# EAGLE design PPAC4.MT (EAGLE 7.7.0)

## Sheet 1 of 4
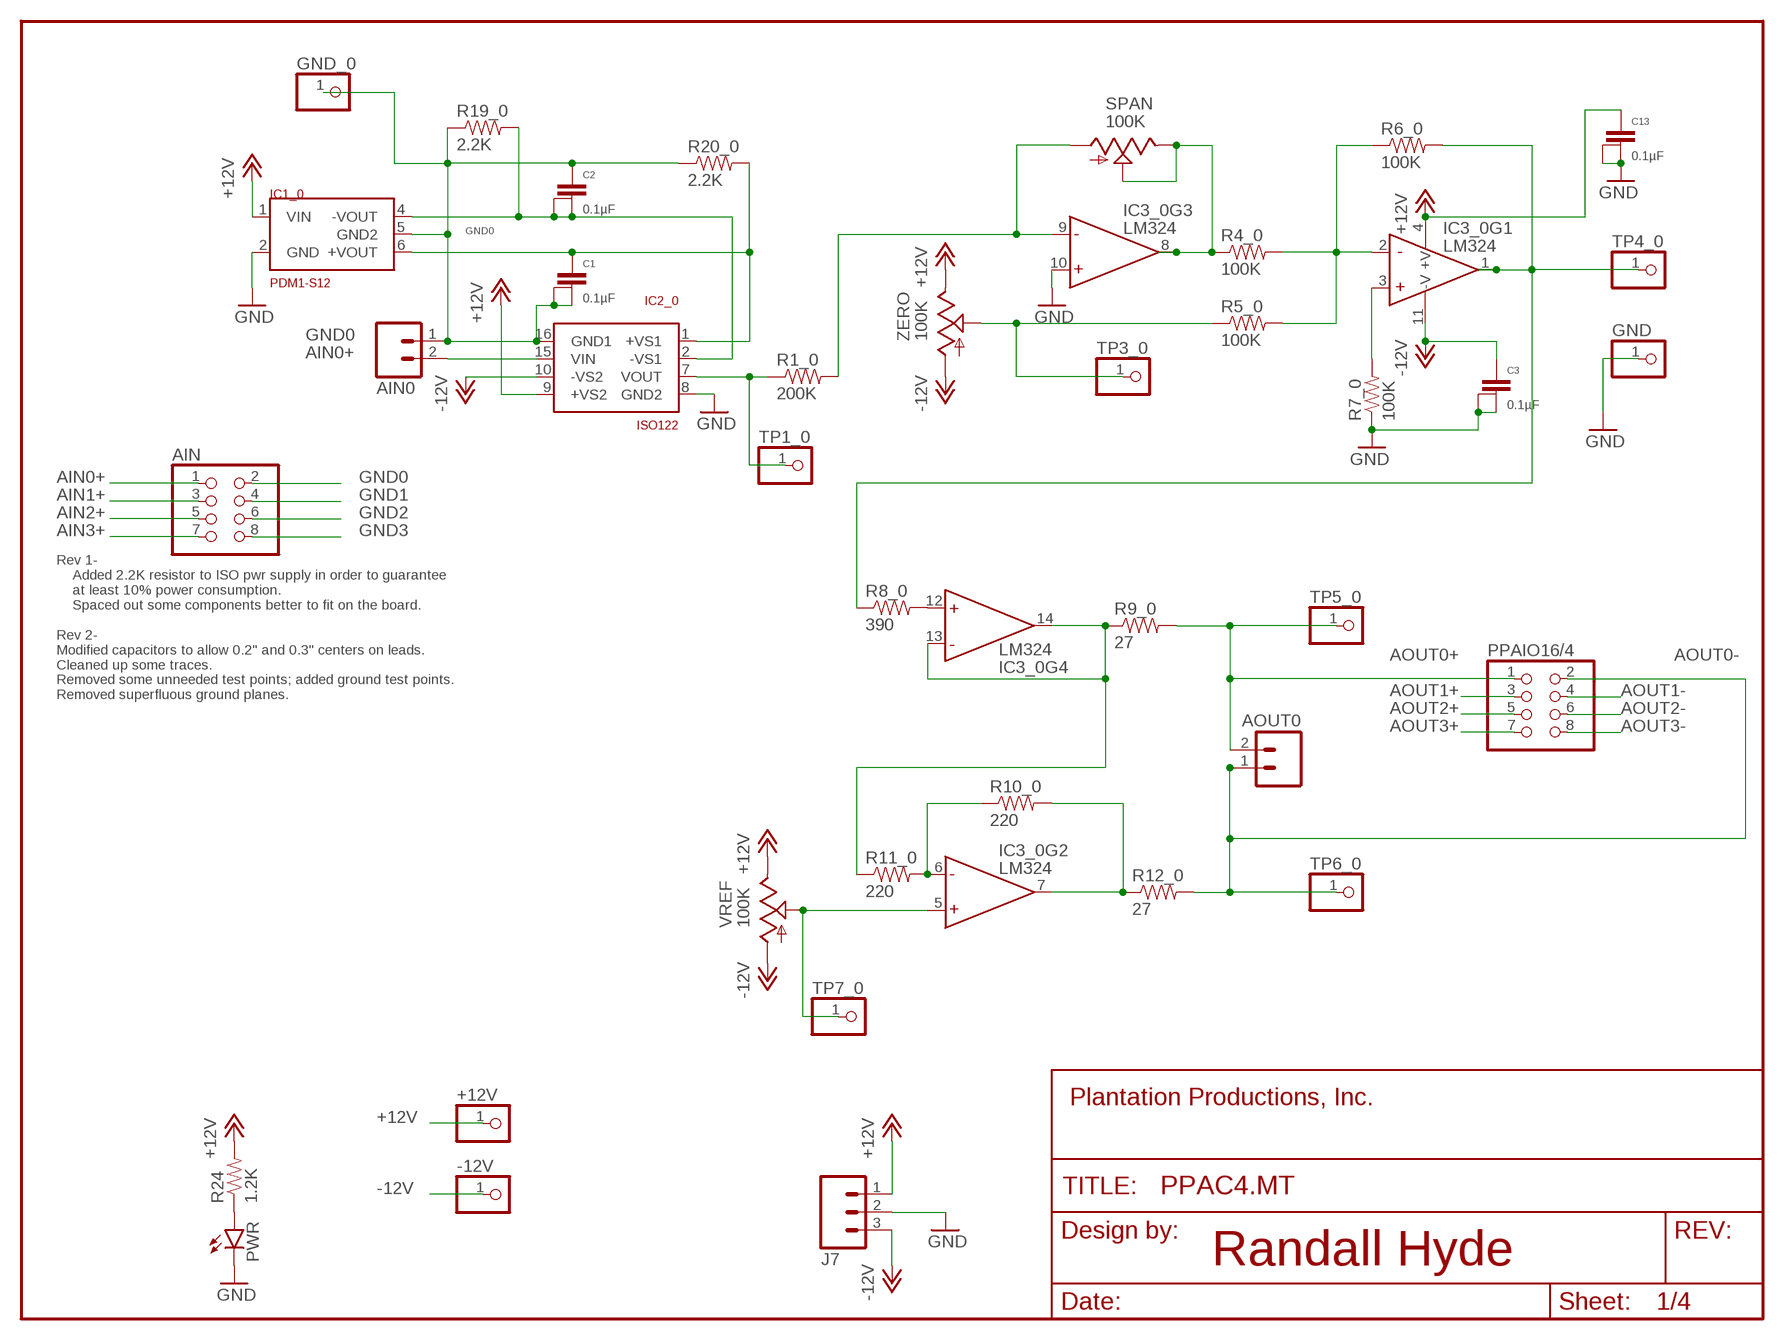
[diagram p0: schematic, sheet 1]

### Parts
+12V  PINHD-1X1  [1X01]
-12V  PINHD-1X1  [1X01]
AIN  PINHD-2X4  [2X04]
AIN0  M025MM  [SCREWTERMINAL-5MM-2]
AOUT0  M025MM  [SCREWTERMINAL-5MM-2]
C1  0.1µF  CAPACITOR  [1+2CAP]
C2  0.1µF  CAPACITOR  [1+2CAP]
C3  0.1µF  CAPACITOR  [1+2CAP]
C13  0.1µF  CAPACITOR  [1+2CAP]
FRAME1  FRAME-LETTERNO_PACKAGE  [DUMMY]
GND  PINHD-1X1  [1X01]
GND_0  PINHD-1X1  [1X01]
IC1_0  PDM1-S12  [SIL6-5]
IC2_0  ISO122  [DIL16-8]
IC3_0  LM324  [DIL14]
J7  M03-SCREW-5MM  [SCREWTERMINAL-5MM-3]
PPAIO16/4  PINHD-2X4  [2X04]
PWR  LED5MM  [LED5MM]
R1_0  200K  10OHM-1/4W-5%(PTH)  [AXIAL-0.3]
R4_0  100K  10OHM-1/4W-5%(PTH)  [AXIAL-0.3]
R5_0  100K  10OHM-1/4W-5%(PTH)  [AXIAL-0.3]
R6_0  100K  10OHM-1/4W-5%(PTH)  [AXIAL-0.3]
R7_0  100K  10OHM-1/4W-5%(PTH)  [AXIAL-0.3]
R8_0  390  10OHM-1/4W-5%(PTH)  [AXIAL-0.3]
R9_0  27  10OHM-1/4W-5%(PTH)  [AXIAL-0.3]
R10_0  220  10OHM-1/4W-5%(PTH)  [AXIAL-0.3]
R11_0  220  10OHM-1/4W-5%(PTH)  [AXIAL-0.3]
R12_0  27  10OHM-1/4W-5%(PTH)  [AXIAL-0.3]
R19_0  2.2K  1KOHM-1/4W-1%(PTH)  [AXIAL-0.3]
R20_0  2.2K  1KOHM-1/4W-1%(PTH)  [AXIAL-0.3]
R24  1.2K  1KOHM-1/4W-1%(PTH)  [AXIAL-0.3]
SPAN  100K  TRIM_US-B64Y  [B64Y]
TP1_0  PINHD-1X1  [1X01]
TP3_0  PINHD-1X1  [1X01]
TP4_0  PINHD-1X1  [1X01]
TP5_0  PINHD-1X1  [1X01]
TP6_0  PINHD-1X1  [1X01]
TP7_0  PINHD-1X1  [1X01]
VREF  100K  TRIM_US-B64Y  [B64Y]
ZERO  100K  TRIM_US-B64Y  [B64Y]

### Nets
+12_0 [RelayConn]: C1.1 IC1_0.6(+VOUT) IC2_0.1(+VS1) R20_0.P$2
+12V: +12V.1 C13.1 IC1_0.1(VIN) IC2_0.9(+VS2) IC3_0.4(+V) J7.1 R24.P$2 VREF.E ZERO.E ; also sheet 2,3,4
-12_0 [RelayConn]: C2.2@1 C2.2@2 IC1_0.4(-VOUT) IC2_0.2(-VS1) R19_0.P$2
-12V [RelayConn]: -12V.1 C3.1 IC2_0.10(-VS2) IC3_0.11(-V) J7.3 VREF.A ZERO.A ; also sheet 2,3,4
AIN0+: AIN0.2 AIN.1 IC2_0.15(VIN)
AIN1+: AIN.3 ; also sheet 2
AIN2+: AIN.5 ; also sheet 3
AIN3+: AIN.7 ; also sheet 4
AOUT0+: AOUT0.2 PPAIO16/4.1 R9_0.P$2 TP5_0.1
AOUT0-: AOUT0.1 PPAIO16/4.2 R12_0.P$2 TP6_0.1
AOUT1+: PPAIO16/4.3 ; also sheet 2
AOUT1-: PPAIO16/4.4 ; also sheet 2
AOUT2+: PPAIO16/4.5 ; also sheet 3
AOUT2-: PPAIO16/4.6 ; also sheet 3
AOUT3+: PPAIO16/4.7 ; also sheet 4
AOUT3-: PPAIO16/4.8 ; also sheet 4
GND [Ground]: C3.2@1 C3.2@2 C13.2@1 C13.2@2 GND.1 IC1_0.2(GND) IC2_0.8(GND2) IC3_0.10(+IN) J7.2 PWR.K(C) R7_0.P$1 ; also sheet 2,3,4
GND0: AIN0.1 AIN.2 C1.2@1 C1.2@2 C2.1 GND_0.1 IC1_0.5(GND2) IC2_0.16(GND1) R19_0.P$1 R20_0.P$1
GND1: AIN.4 ; also sheet 2
GND2: AIN.6 ; also sheet 3
GND3: AIN.8 ; also sheet 4
N$1: IC3_0.9(-IN) R1_0.P$2 SPAN.A
N$2: IC3_0.3(+IN) R7_0.P$2
N$3: IC3_0.8(OUT) R4_0.P$1 SPAN.E SPAN.S
N$4: IC3_0.2(-IN) R4_0.P$2 R5_0.P$2 R6_0.P$1
N$5: IC3_0.1(OUT) R6_0.P$2 R8_0.P$1 TP4_0.1
N$6: R5_0.P$1 TP3_0.1 ZERO.S
N$8: IC2_0.7(VOUT) R1_0.P$1 TP1_0.1
N$9: IC3_0.12(+IN) R8_0.P$2
N$10: IC3_0.7(OUT) R10_0.P$2 R12_0.P$1
N$11: IC3_0.13(-IN) IC3_0.14(OUT) R9_0.P$1 R11_0.P$1
N$12: IC3_0.6(-IN) R10_0.P$1 R11_0.P$2
N$13: IC3_0.5(+IN) TP7_0.1 VREF.S
N$26: PWR.A R24.P$1

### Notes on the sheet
- Rev 1-
      Added 2.2K resistor to ISO pwr supply in order to guarantee
      at least 10% power consumption.
      Spaced out some components better to fit on the board.
  
  Rev 2-
  Modified capacitors to allow 0.2" and 0.3" centers on leads.
  Cleaned up some traces.
  Removed some unneeded test points; added ground test points.
  Removed superfluous ground planes.
- Randall Hyde

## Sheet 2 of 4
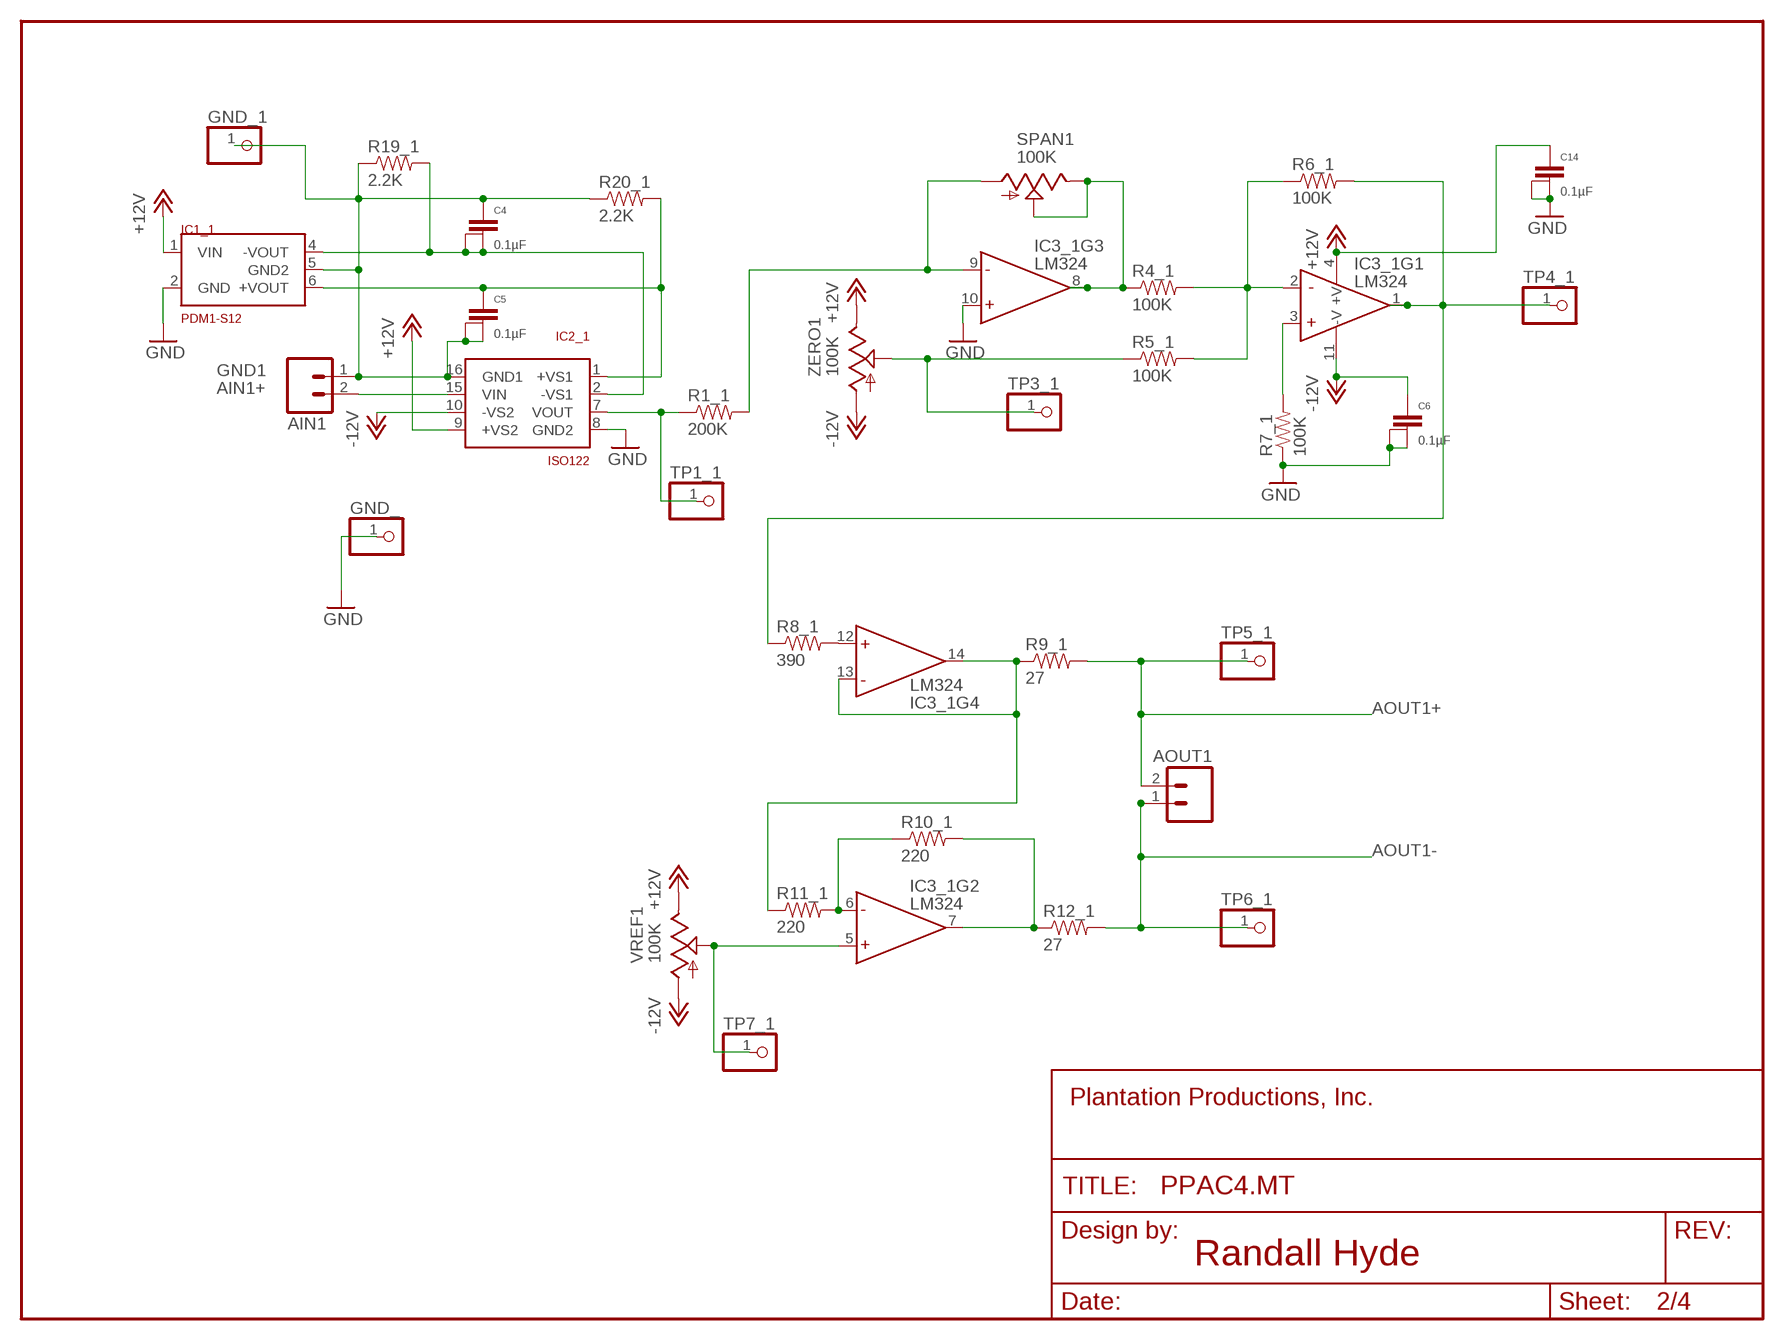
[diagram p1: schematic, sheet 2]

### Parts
AIN1  M025MM  [SCREWTERMINAL-5MM-2]
AOUT1  M025MM  [SCREWTERMINAL-5MM-2]
C4  0.1µF  CAPACITOR  [1+2CAP]
C5  0.1µF  CAPACITOR  [1+2CAP]
C6  0.1µF  CAPACITOR  [1+2CAP]
C14  0.1µF  CAPACITOR  [1+2CAP]
FRAME2  FRAME-LETTERNO_PACKAGE  [DUMMY]
GND_  PINHD-1X1  [1X01]
GND_1  PINHD-1X1  [1X01]
IC1_1  PDM1-S12  [SIL6-5]
IC2_1  ISO122  [DIL16-8]
IC3_1  LM324  [DIL14]
R1_1  200K  10OHM-1/4W-5%(PTH)  [AXIAL-0.3]
R4_1  100K  10OHM-1/4W-5%(PTH)  [AXIAL-0.3]
R5_1  100K  10OHM-1/4W-5%(PTH)  [AXIAL-0.3]
R6_1  100K  10OHM-1/4W-5%(PTH)  [AXIAL-0.3]
R7_1  100K  10OHM-1/4W-5%(PTH)  [AXIAL-0.3]
R8_1  390  10OHM-1/4W-5%(PTH)  [AXIAL-0.3]
R9_1  27  10OHM-1/4W-5%(PTH)  [AXIAL-0.3]
R10_1  220  10OHM-1/4W-5%(PTH)  [AXIAL-0.3]
R11_1  220  10OHM-1/4W-5%(PTH)  [AXIAL-0.3]
R12_1  27  10OHM-1/4W-5%(PTH)  [AXIAL-0.3]
R19_1  2.2K  1KOHM-1/4W-1%(PTH)  [AXIAL-0.3]
R20_1  2.2K  1KOHM-1/4W-1%(PTH)  [AXIAL-0.3]
SPAN1  100K  TRIM_US-B64Y  [B64Y]
TP1_1  PINHD-1X1  [1X01]
TP3_1  PINHD-1X1  [1X01]
TP4_1  PINHD-1X1  [1X01]
TP5_1  PINHD-1X1  [1X01]
TP6_1  PINHD-1X1  [1X01]
TP7_1  PINHD-1X1  [1X01]
VREF1  100K  TRIM_US-B64Y  [B64Y]
ZERO1  100K  TRIM_US-B64Y  [B64Y]

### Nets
+12_1 [RelayConn]: C5.1 IC1_1.6(+VOUT) IC2_1.1(+VS1) R20_1.P$2
+12V: C14.1 IC1_1.1(VIN) IC2_1.9(+VS2) IC3_1.4(+V) VREF1.E ZERO1.E ; also sheet 1,3,4
-12_1 [RelayConn]: C4.2@1 C4.2@2 IC1_1.4(-VOUT) IC2_1.2(-VS1) R19_1.P$2
-12V [RelayConn]: C6.1 IC2_1.10(-VS2) IC3_1.11(-V) VREF1.A ZERO1.A ; also sheet 1,3,4
AIN1+: AIN1.2 IC2_1.15(VIN) ; also sheet 1
AOUT1+: AOUT1.2 R9_1.P$2 TP5_1.1 ; also sheet 1
AOUT1-: AOUT1.1 R12_1.P$2 TP6_1.1 ; also sheet 1
GND [Ground]: C6.2@1 C6.2@2 C14.2@1 C14.2@2 GND_.1 IC1_1.2(GND) IC2_1.8(GND2) IC3_1.10(+IN) R7_1.P$1 ; also sheet 1,3,4
GND1: AIN1.1 C4.1 C5.2@1 C5.2@2 GND_1.1 IC1_1.5(GND2) IC2_1.16(GND1) R19_1.P$1 R20_1.P$1 ; also sheet 1
N$17: IC3_1.9(-IN) R1_1.P$2 SPAN1.A
N$18: IC3_1.8(OUT) R4_1.P$1 SPAN1.E SPAN1.S
N$19: IC3_1.2(-IN) R4_1.P$2 R5_1.P$2 R6_1.P$1
N$20: IC3_1.1(OUT) R6_1.P$2 R8_1.P$1 TP4_1.1
N$22: IC2_1.7(VOUT) R1_1.P$1 TP1_1.1
N$23: R5_1.P$1 TP3_1.1 ZERO1.S
N$24: IC3_1.3(+IN) R7_1.P$2
N$29: IC3_1.7(OUT) R10_1.P$2 R12_1.P$1
N$30: IC3_1.12(+IN) R8_1.P$2
N$31: IC3_1.13(-IN) IC3_1.14(OUT) R9_1.P$1 R11_1.P$1
N$32: IC3_1.6(-IN) R10_1.P$1 R11_1.P$2
N$33: IC3_1.5(+IN) TP7_1.1 VREF1.S

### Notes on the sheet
- Randall Hyde

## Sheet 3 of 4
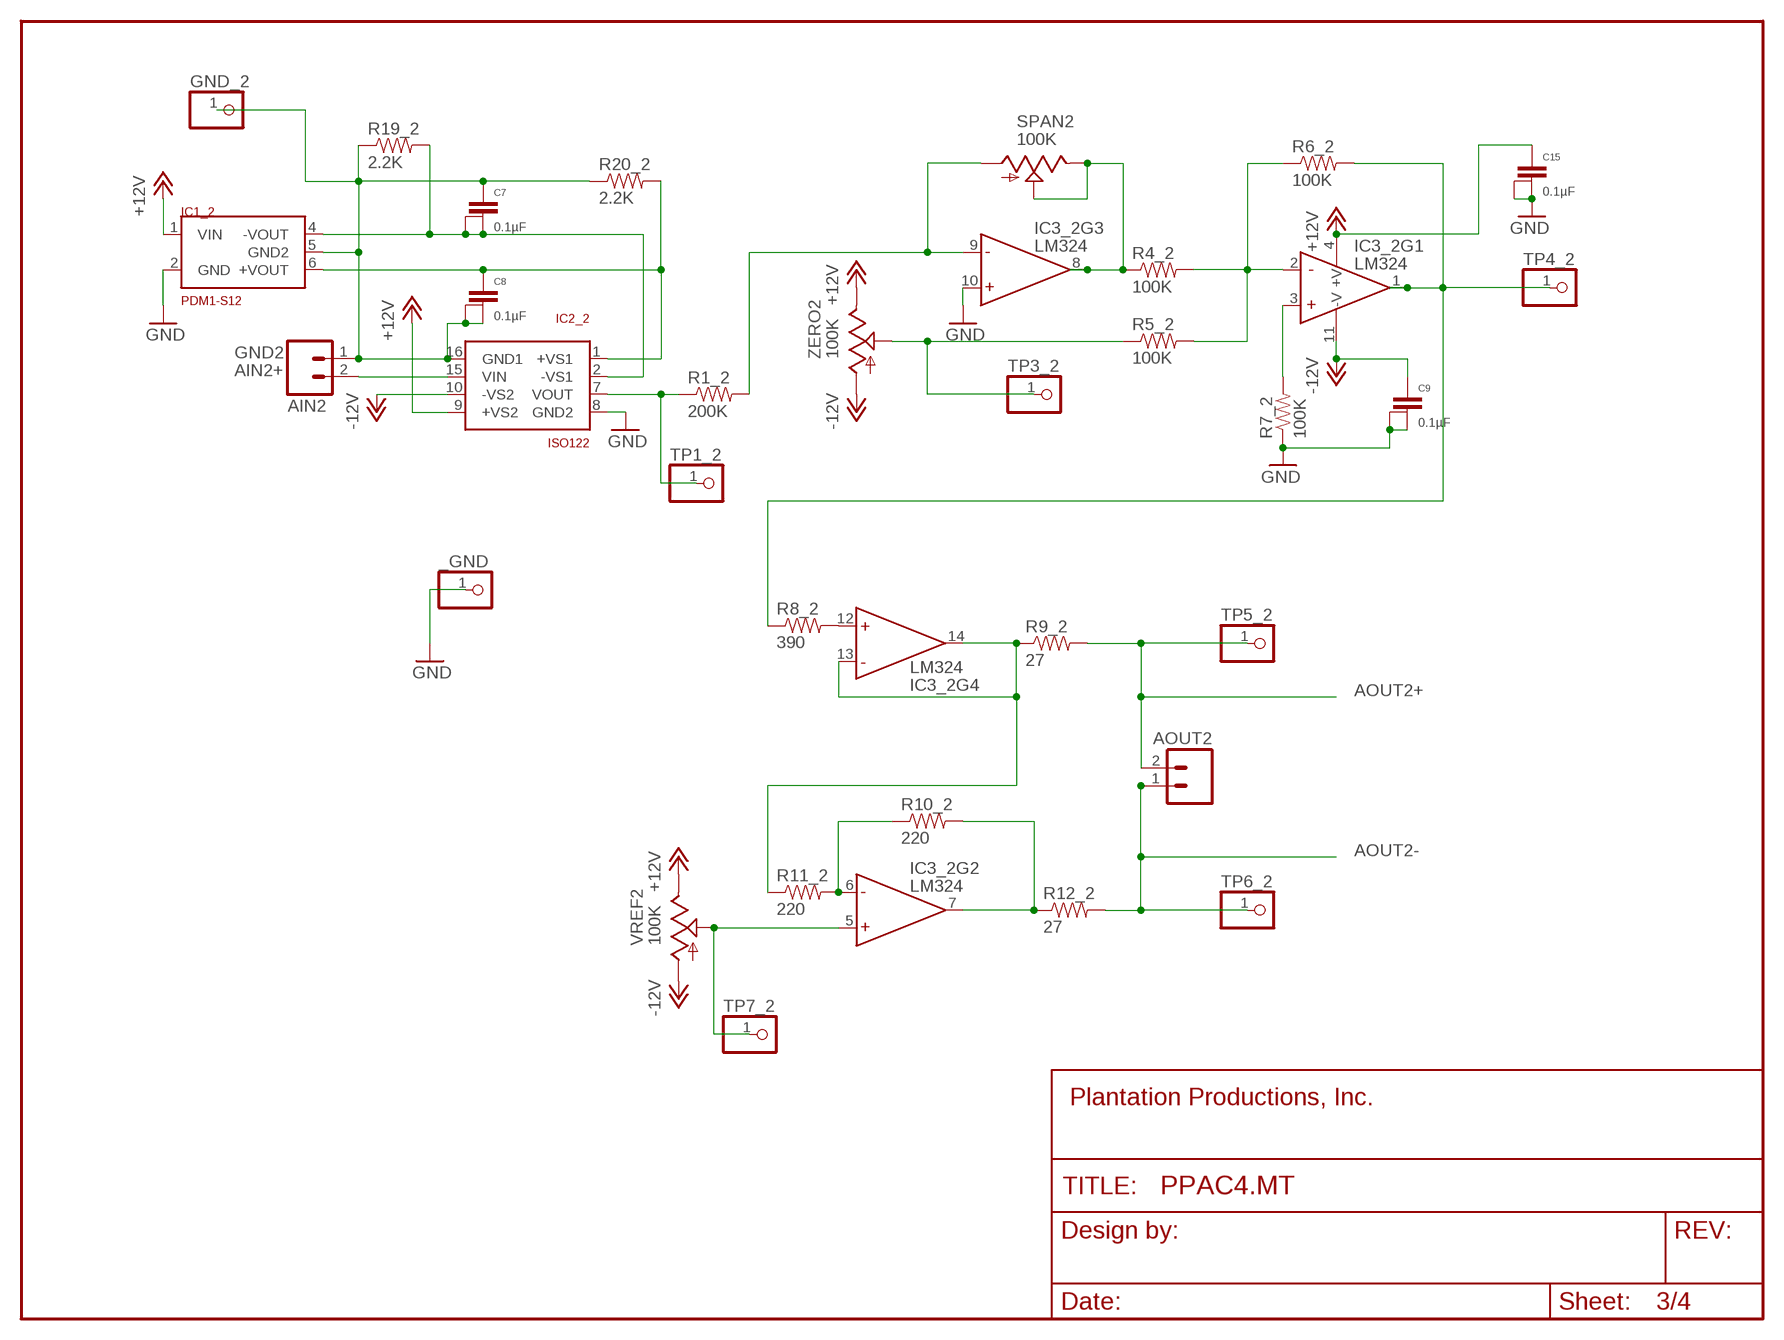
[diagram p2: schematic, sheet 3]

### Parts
_GND  PINHD-1X1  [1X01]
AIN2  M025MM  [SCREWTERMINAL-5MM-2]
AOUT2  M025MM  [SCREWTERMINAL-5MM-2]
C7  0.1µF  CAPACITOR  [1+2CAP]
C8  0.1µF  CAPACITOR  [1+2CAP]
C9  0.1µF  CAPACITOR  [1+2CAP]
C15  0.1µF  CAPACITOR  [1+2CAP]
FRAME3  FRAME-LETTERNO_PACKAGE  [DUMMY]
GND_2  PINHD-1X1  [1X01]
IC1_2  PDM1-S12  [SIL6-5]
IC2_2  ISO122  [DIL16-8]
IC3_2  LM324  [DIL14]
R1_2  200K  10OHM-1/4W-5%(PTH)  [AXIAL-0.3]
R4_2  100K  10OHM-1/4W-5%(PTH)  [AXIAL-0.3]
R5_2  100K  10OHM-1/4W-5%(PTH)  [AXIAL-0.3]
R6_2  100K  10OHM-1/4W-5%(PTH)  [AXIAL-0.3]
R7_2  100K  10OHM-1/4W-5%(PTH)  [AXIAL-0.3]
R8_2  390  10OHM-1/4W-5%(PTH)  [AXIAL-0.3]
R9_2  27  10OHM-1/4W-5%(PTH)  [AXIAL-0.3]
R10_2  220  10OHM-1/4W-5%(PTH)  [AXIAL-0.3]
R11_2  220  10OHM-1/4W-5%(PTH)  [AXIAL-0.3]
R12_2  27  10OHM-1/4W-5%(PTH)  [AXIAL-0.3]
R19_2  2.2K  1KOHM-1/4W-1%(PTH)  [AXIAL-0.3]
R20_2  2.2K  1KOHM-1/4W-1%(PTH)  [AXIAL-0.3]
SPAN2  100K  TRIM_US-B64Y  [B64Y]
TP1_2  PINHD-1X1  [1X01]
TP3_2  PINHD-1X1  [1X01]
TP4_2  PINHD-1X1  [1X01]
TP5_2  PINHD-1X1  [1X01]
TP6_2  PINHD-1X1  [1X01]
TP7_2  PINHD-1X1  [1X01]
VREF2  100K  TRIM_US-B64Y  [B64Y]
ZERO2  100K  TRIM_US-B64Y  [B64Y]

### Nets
+12_2 [RelayConn]: C8.1 IC1_2.6(+VOUT) IC2_2.1(+VS1) R20_2.P$2
+12V: C15.1 IC1_2.1(VIN) IC2_2.9(+VS2) IC3_2.4(+V) VREF2.E ZERO2.E ; also sheet 1,2,4
-12_2 [RelayConn]: C7.2@1 C7.2@2 IC1_2.4(-VOUT) IC2_2.2(-VS1) R19_2.P$2
-12V [RelayConn]: C9.1 IC2_2.10(-VS2) IC3_2.11(-V) VREF2.A ZERO2.A ; also sheet 1,2,4
AIN2+: AIN2.2 IC2_2.15(VIN) ; also sheet 1
AOUT2+: AOUT2.2 R9_2.P$2 TP5_2.1 ; also sheet 1
AOUT2-: AOUT2.1 R12_2.P$2 TP6_2.1 ; also sheet 1
GND [Ground]: _GND.1 C9.2@1 C9.2@2 C15.2@1 C15.2@2 IC1_2.2(GND) IC2_2.8(GND2) IC3_2.10(+IN) R7_2.P$1 ; also sheet 1,2,4
GND2: AIN2.1 C7.1 C8.2@1 C8.2@2 GND_2.1 IC1_2.5(GND2) IC2_2.16(GND1) R19_2.P$1 R20_2.P$1 ; also sheet 1
N$34: IC3_2.9(-IN) R1_2.P$2 SPAN2.A
N$35: IC3_2.8(OUT) R4_2.P$1 SPAN2.E SPAN2.S
N$36: IC3_2.2(-IN) R4_2.P$2 R5_2.P$2 R6_2.P$1
N$37: IC3_2.1(OUT) R6_2.P$2 R8_2.P$1 TP4_2.1
N$39: IC2_2.7(VOUT) R1_2.P$1 TP1_2.1
N$40: R5_2.P$1 TP3_2.1 ZERO2.S
N$41: IC3_2.3(+IN) R7_2.P$2
N$45: IC3_2.7(OUT) R10_2.P$2 R12_2.P$1
N$46: IC3_2.12(+IN) R8_2.P$2
N$47: IC3_2.13(-IN) IC3_2.14(OUT) R9_2.P$1 R11_2.P$1
N$48: IC3_2.6(-IN) R10_2.P$1 R11_2.P$2
N$49: IC3_2.5(+IN) TP7_2.1 VREF2.S

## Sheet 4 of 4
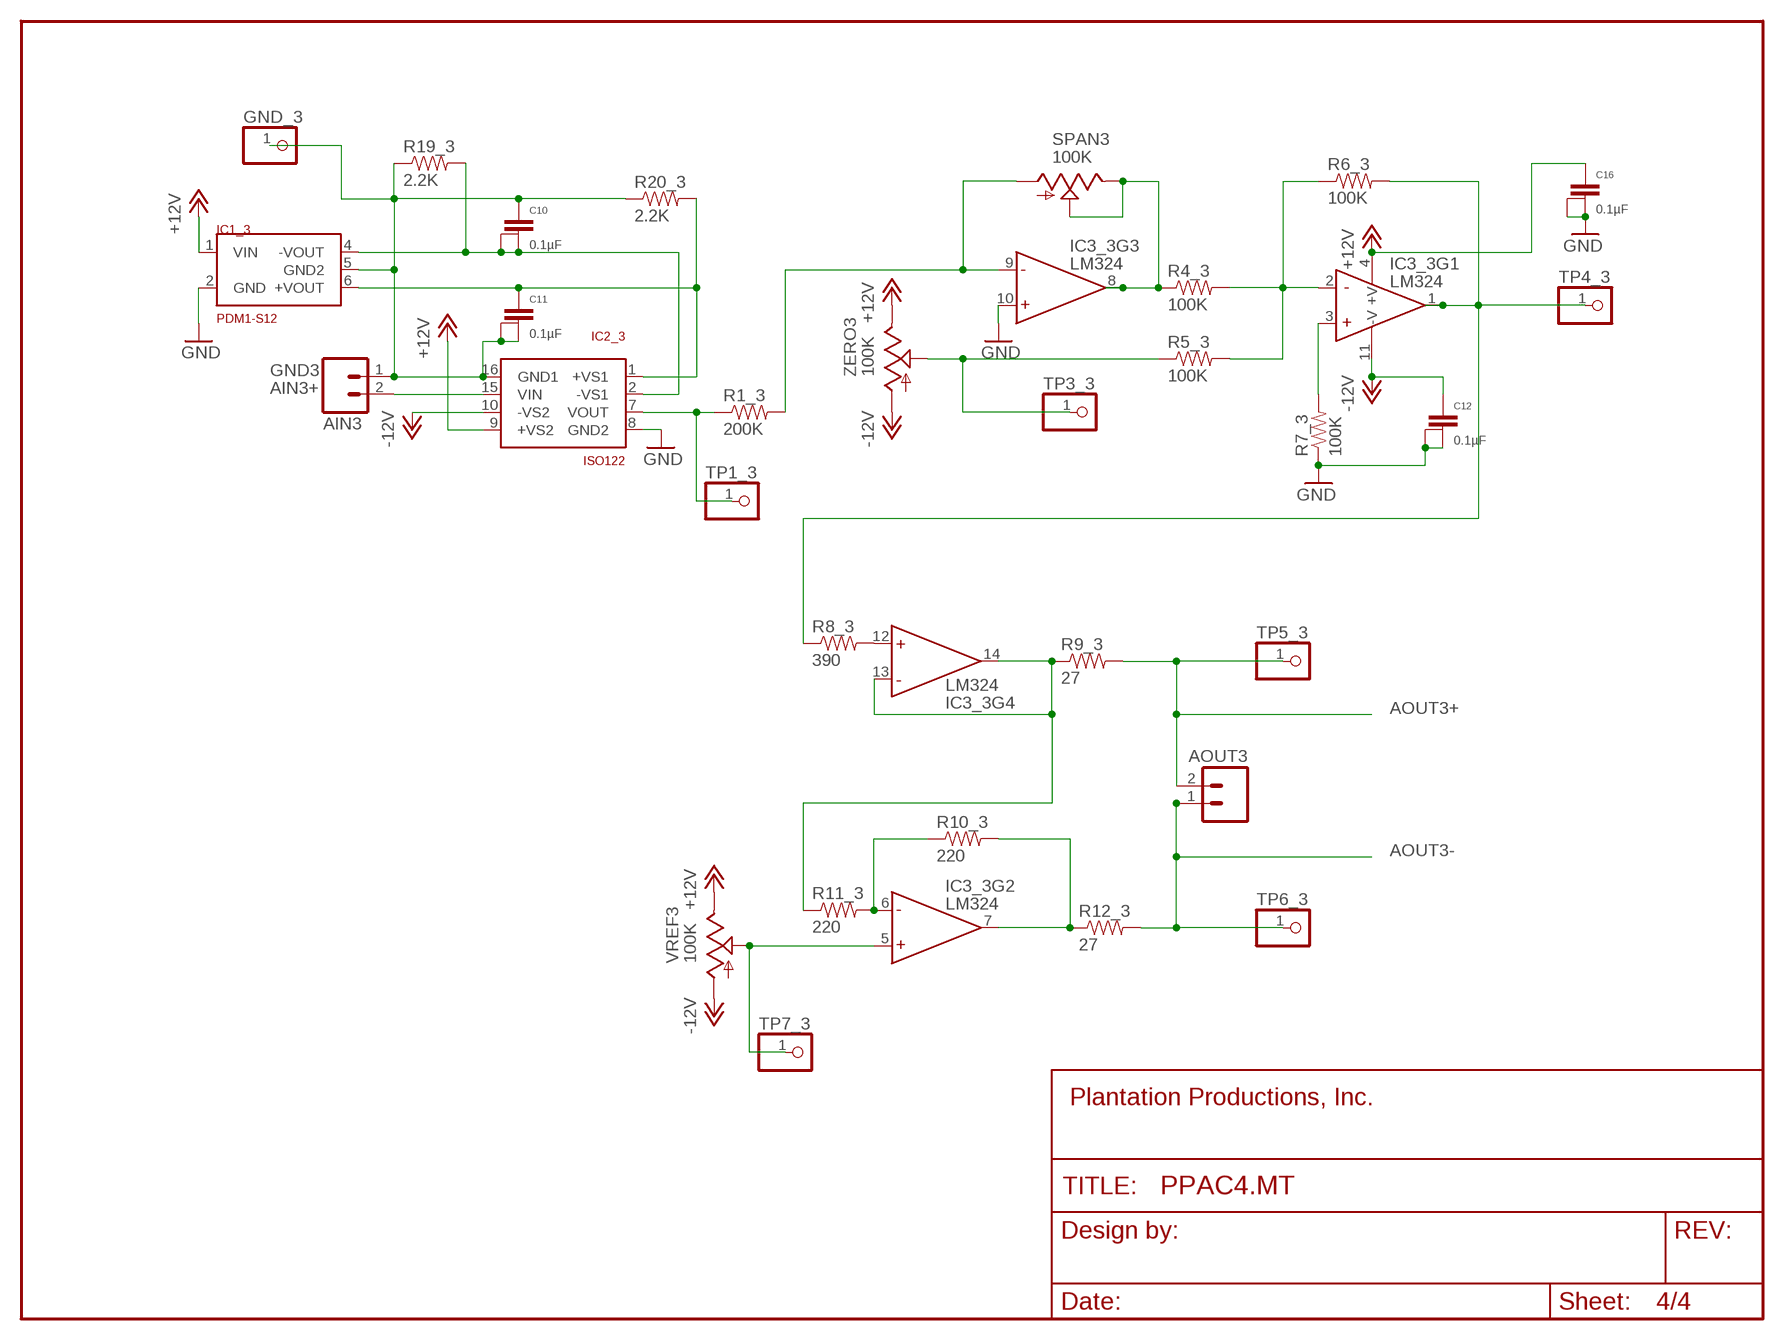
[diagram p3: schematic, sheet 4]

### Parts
AIN3  M025MM  [SCREWTERMINAL-5MM-2]
AOUT3  M025MM  [SCREWTERMINAL-5MM-2]
C10  0.1µF  CAPACITOR  [1+2CAP]
C11  0.1µF  CAPACITOR  [1+2CAP]
C12  0.1µF  CAPACITOR  [1+2CAP]
C16  0.1µF  CAPACITOR  [1+2CAP]
FRAME4  FRAME-LETTERNO_PACKAGE  [DUMMY]
GND_3  PINHD-1X1  [1X01]
IC1_3  PDM1-S12  [SIL6-5]
IC2_3  ISO122  [DIL16-8]
IC3_3  LM324  [DIL14]
R1_3  200K  10OHM-1/4W-5%(PTH)  [AXIAL-0.3]
R4_3  100K  10OHM-1/4W-5%(PTH)  [AXIAL-0.3]
R5_3  100K  10OHM-1/4W-5%(PTH)  [AXIAL-0.3]
R6_3  100K  10OHM-1/4W-5%(PTH)  [AXIAL-0.3]
R7_3  100K  10OHM-1/4W-5%(PTH)  [AXIAL-0.3]
R8_3  390  10OHM-1/4W-5%(PTH)  [AXIAL-0.3]
R9_3  27  10OHM-1/4W-5%(PTH)  [AXIAL-0.3]
R10_3  220  10OHM-1/4W-5%(PTH)  [AXIAL-0.3]
R11_3  220  10OHM-1/4W-5%(PTH)  [AXIAL-0.3]
R12_3  27  10OHM-1/4W-5%(PTH)  [AXIAL-0.3]
R19_3  2.2K  1KOHM-1/4W-1%(PTH)  [AXIAL-0.3]
R20_3  2.2K  1KOHM-1/4W-1%(PTH)  [AXIAL-0.3]
SPAN3  100K  TRIM_US-B64Y  [B64Y]
TP1_3  PINHD-1X1  [1X01]
TP3_3  PINHD-1X1  [1X01]
TP4_3  PINHD-1X1  [1X01]
TP5_3  PINHD-1X1  [1X01]
TP6_3  PINHD-1X1  [1X01]
TP7_3  PINHD-1X1  [1X01]
VREF3  100K  TRIM_US-B64Y  [B64Y]
ZERO3  100K  TRIM_US-B64Y  [B64Y]

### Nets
+12_3 [RelayConn]: C11.1 IC1_3.6(+VOUT) IC2_3.1(+VS1) R20_3.P$2
+12V: C16.1 IC1_3.1(VIN) IC2_3.9(+VS2) IC3_3.4(+V) VREF3.E ZERO3.E ; also sheet 1,2,3
-12_3 [RelayConn]: C10.2@1 C10.2@2 IC1_3.4(-VOUT) IC2_3.2(-VS1) R19_3.P$2
-12V [RelayConn]: C12.1 IC2_3.10(-VS2) IC3_3.11(-V) VREF3.A ZERO3.A ; also sheet 1,2,3
AIN3+: AIN3.2 IC2_3.15(VIN) ; also sheet 1
AOUT3+: AOUT3.2 R9_3.P$2 TP5_3.1 ; also sheet 1
AOUT3-: AOUT3.1 R12_3.P$2 TP6_3.1 ; also sheet 1
GND [Ground]: C12.2@1 C12.2@2 C16.2@1 C16.2@2 IC1_3.2(GND) IC2_3.8(GND2) IC3_3.10(+IN) R7_3.P$1 ; also sheet 1,2,3
GND3: AIN3.1 C10.1 C11.2@1 C11.2@2 GND_3.1 IC1_3.5(GND2) IC2_3.16(GND1) R19_3.P$1 R20_3.P$1 ; also sheet 1
N$50: IC3_3.9(-IN) R1_3.P$2 SPAN3.A
N$51: IC3_3.8(OUT) R4_3.P$1 SPAN3.E SPAN3.S
N$52: IC3_3.2(-IN) R4_3.P$2 R5_3.P$2 R6_3.P$1
N$53: IC3_3.1(OUT) R6_3.P$2 R8_3.P$1 TP4_3.1
N$55: IC2_3.7(VOUT) R1_3.P$1 TP1_3.1
N$56: R5_3.P$1 TP3_3.1 ZERO3.S
N$57: IC3_3.3(+IN) R7_3.P$2
N$61: IC3_3.7(OUT) R10_3.P$2 R12_3.P$1
N$62: IC3_3.12(+IN) R8_3.P$2
N$63: IC3_3.13(-IN) IC3_3.14(OUT) R9_3.P$1 R11_3.P$1
N$64: IC3_3.6(-IN) R10_3.P$1 R11_3.P$2
N$65: IC3_3.5(+IN) TP7_3.1 VREF3.S

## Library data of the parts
+12V -12V _GND GND GND_ GND_0 GND_1-GND_3 TP1_0 TP1_1-TP1_3 TP3_0 TP3_1-TP3_3 TP4_0 TP4_1-TP4_3 TP5_0 TP5_1-TP5_3 TP6_0 TP6_1-TP6_3 TP7_0 TP7_1-TP7_3 = pinhead:PINHD-1X1: PIN HEADER
AIN PPAIO16/4 = pinhead:PINHD-2X4: PIN HEADER
AIN0 AIN1-AIN3 AOUT0 AOUT1-AOUT3 = SparkFun-Connectors:M02: Standard 2-pin 0.1" header. Use with; STOREFRONT_ID: PRT-08432
C1-C16 = PlantProd:CAPACITOR: Capacitor with three terminals to support multiple capacitor sizes.
FRAME1-FRAME4 = SparkFun-Aesthetics:FRAME-LETTER: Schematic Frame; DESIGNER: Nobody; VERSION: v01
IC1_0 IC1_1-IC1_3 = PlantProd:PDM1-S12: PDM1-12S Isolated Power Supply 12V to +/-12V
IC2_0 IC2_1-IC2_3 = PlantProd:ISO122: ISO122 - single channel isolation amplifier
IC3_0 IC3_1-IC3_3 = PlantProd:LM324: LM324 quad op-amp
J7 = SparkFun-Connectors:M03: Header 3 Standard 3-pin 0.1" header. Use with straight break away headers (SKU : PRT-00116), right angle break away headers (PRT-00553), swiss pins (PRT-00743), machine pins (PRT-00117), and female headers (PRT-00115). Molex polarized connector foot print use with SKU : PRT-08232 with associated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; STOREFRONT_ID: PRT-08433
PWR = SparkFun-LED:LED: LEDs
R1_0 R1_1-R1_3 R4_0 R4_1-R4_3 R5_0 R5_1-R5_3 R6_0 R6_1-R6_3 R7_0 R7_1-R7_3 R8_0 R8_1-R8_3 R9_0 R9_1-R9_3 R10_0 R10_1-R10_3 R11_0 R11_1-R11_3 R12_0 R12_1-R12_3 = SparkFun-Resistors:10OHM-1/4W-5%(PTH): RES-10698; PROD_ID: RES-10698; VALUE: 10
R19_0 R19_1-R19_3 R20_0 R20_1-R20_3 R24 = SparkFun-Resistors:1KOHM-1/4W-1%(PTH): RES-12182; PROD_ID: RES-12182; VALUE: 1K
SPAN SPAN1-SPAN3 VREF VREF1-VREF3 ZERO ZERO1-ZERO3 = pot:TRIM_US-: POTENTIOMETER

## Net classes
1 Ground: width 0.762 mm, drill 1 mm, clearance 0.102 mm
2 RelayConn: width 1.016 mm, drill 0.025 mm, clearance 0.508 mm
3 HiCurSignal: width 1.016 mm, drill 0.025 mm, clearance 1.016 mm

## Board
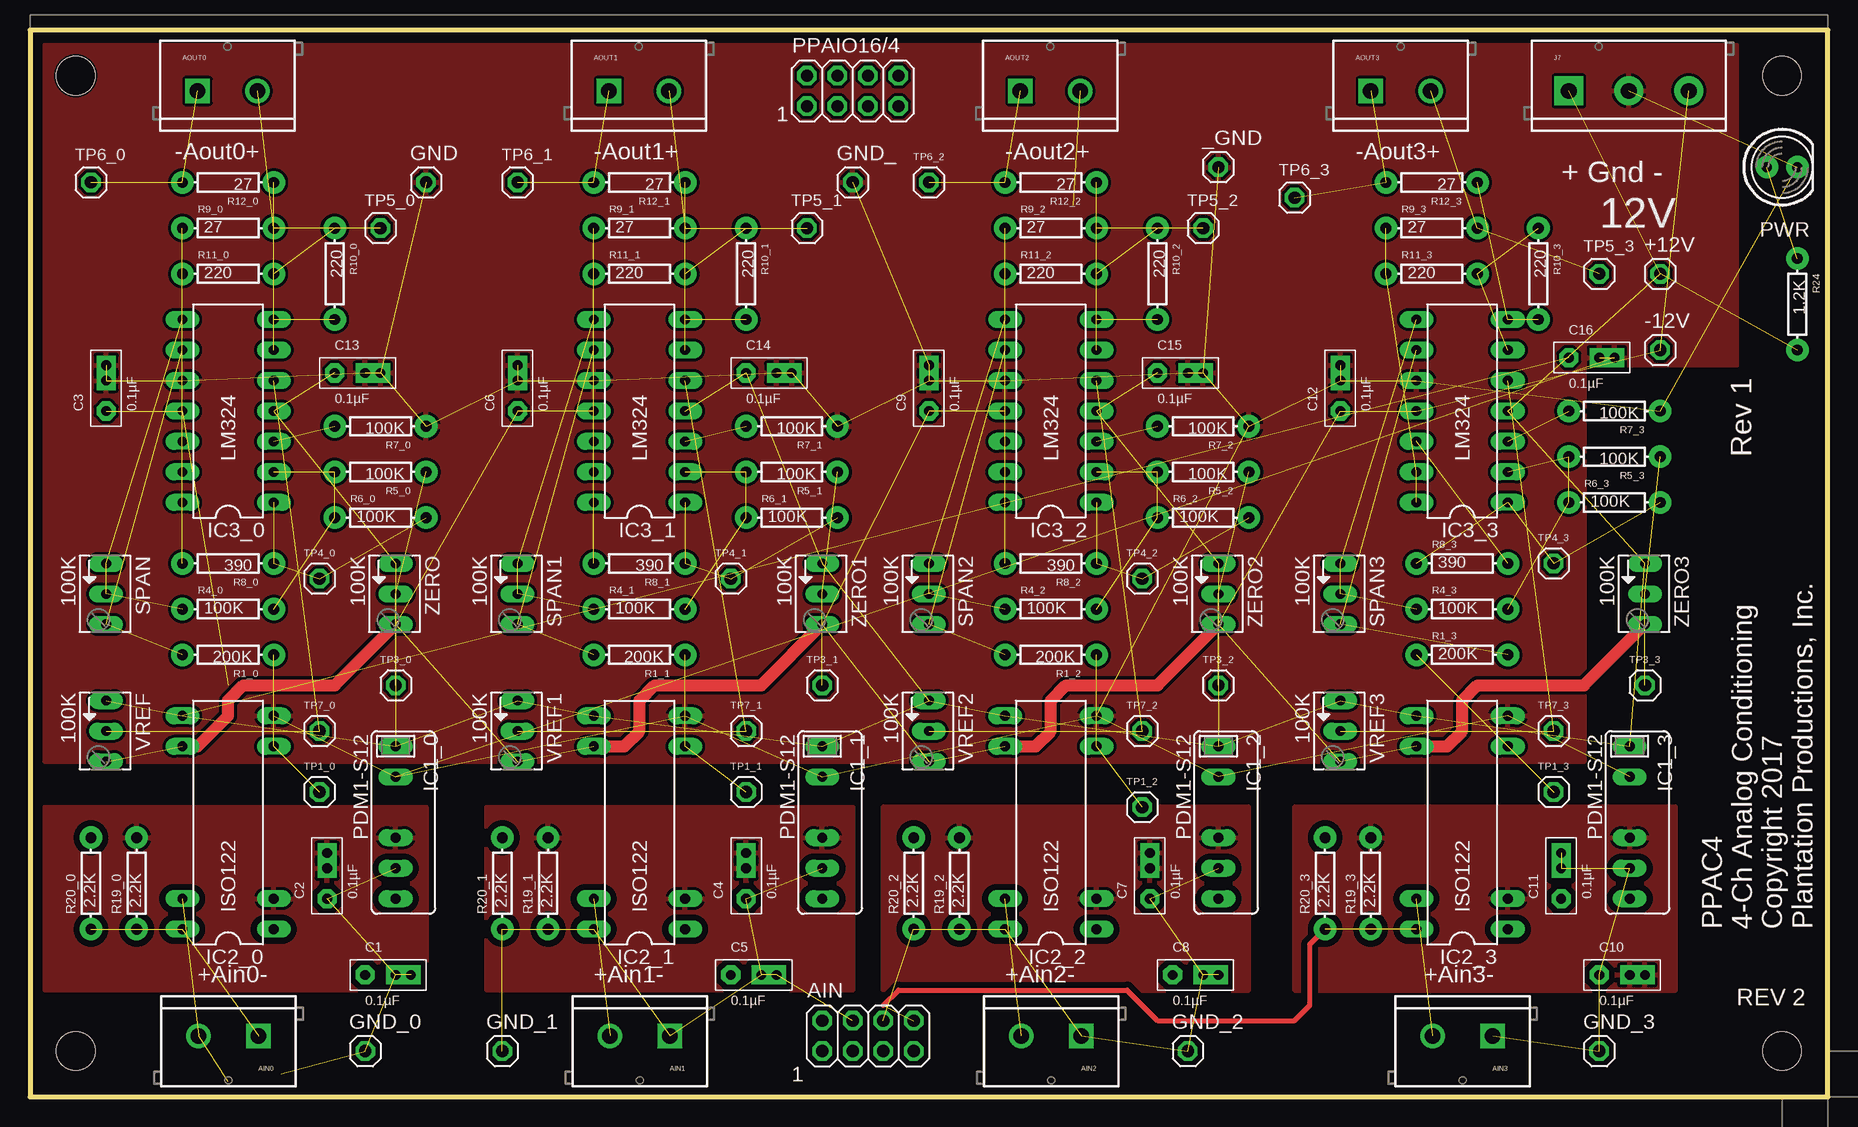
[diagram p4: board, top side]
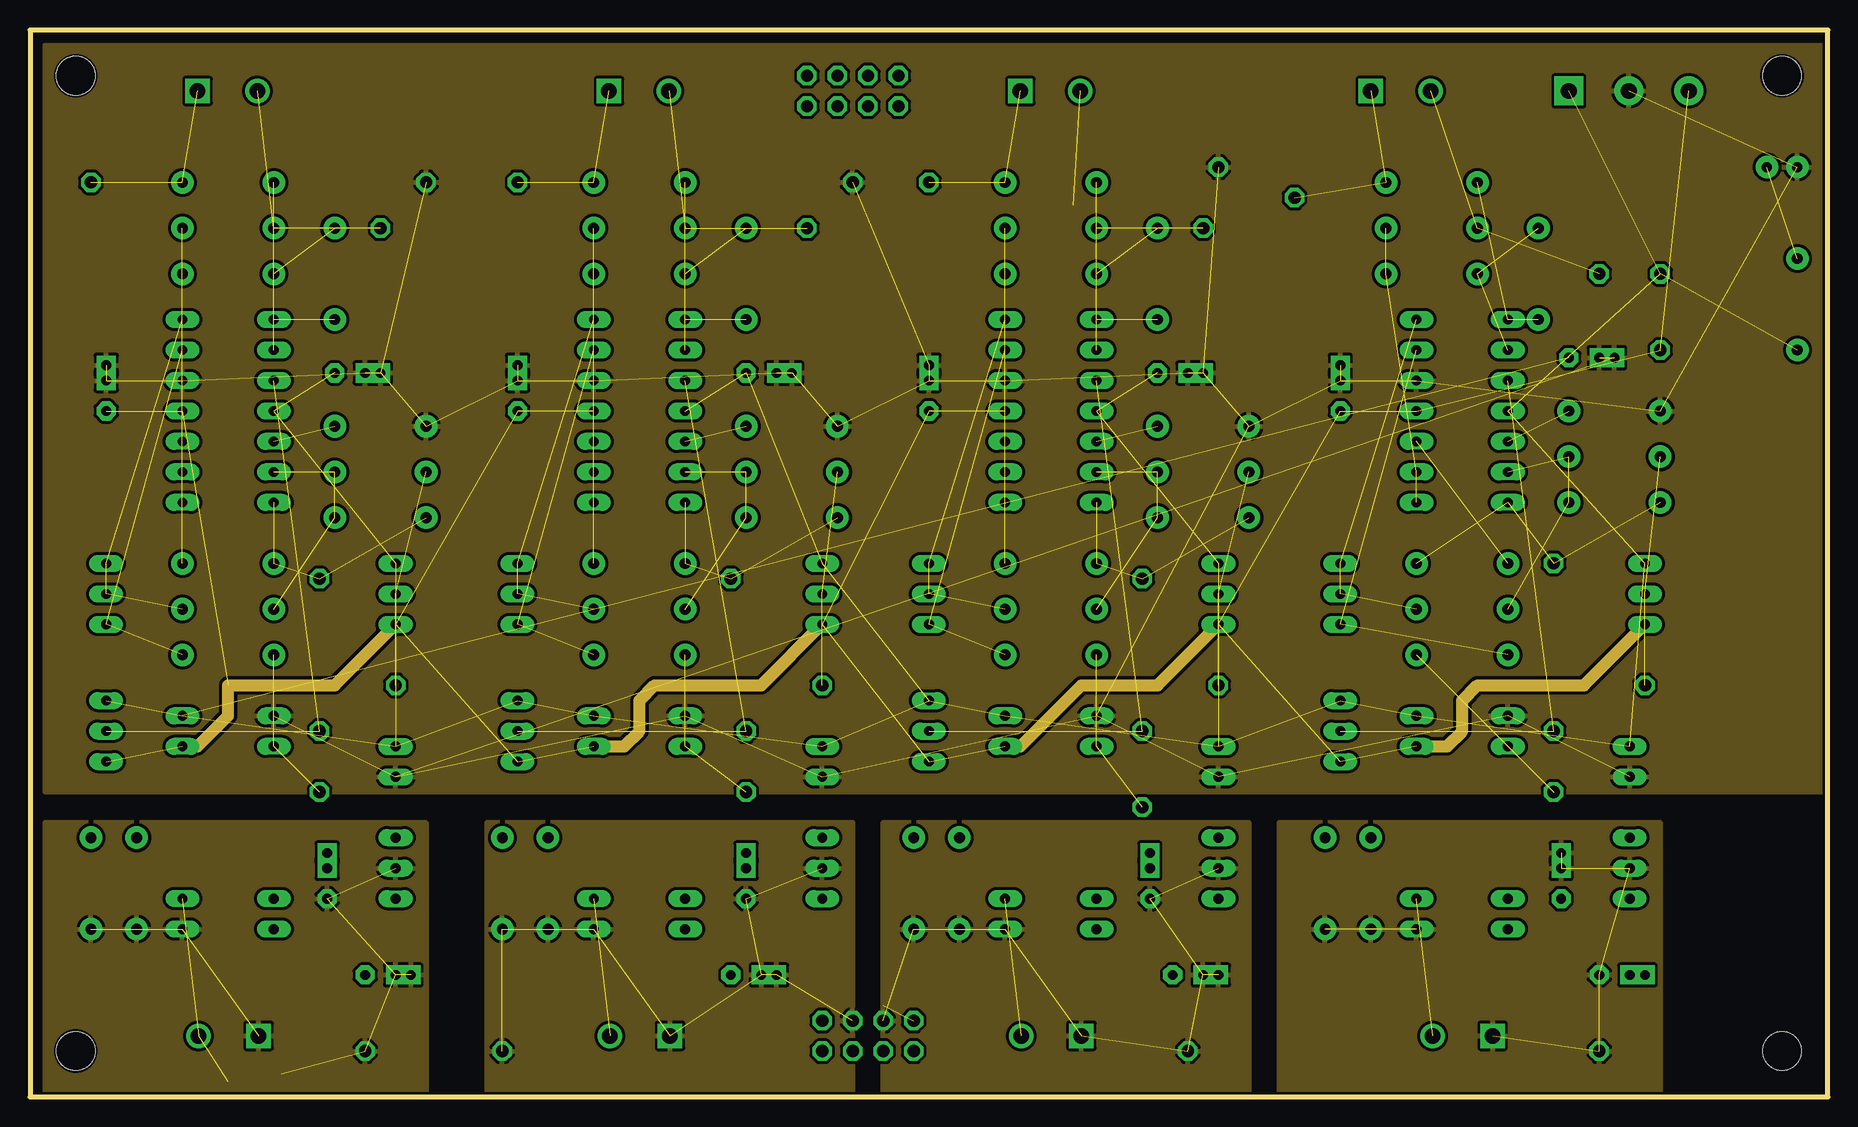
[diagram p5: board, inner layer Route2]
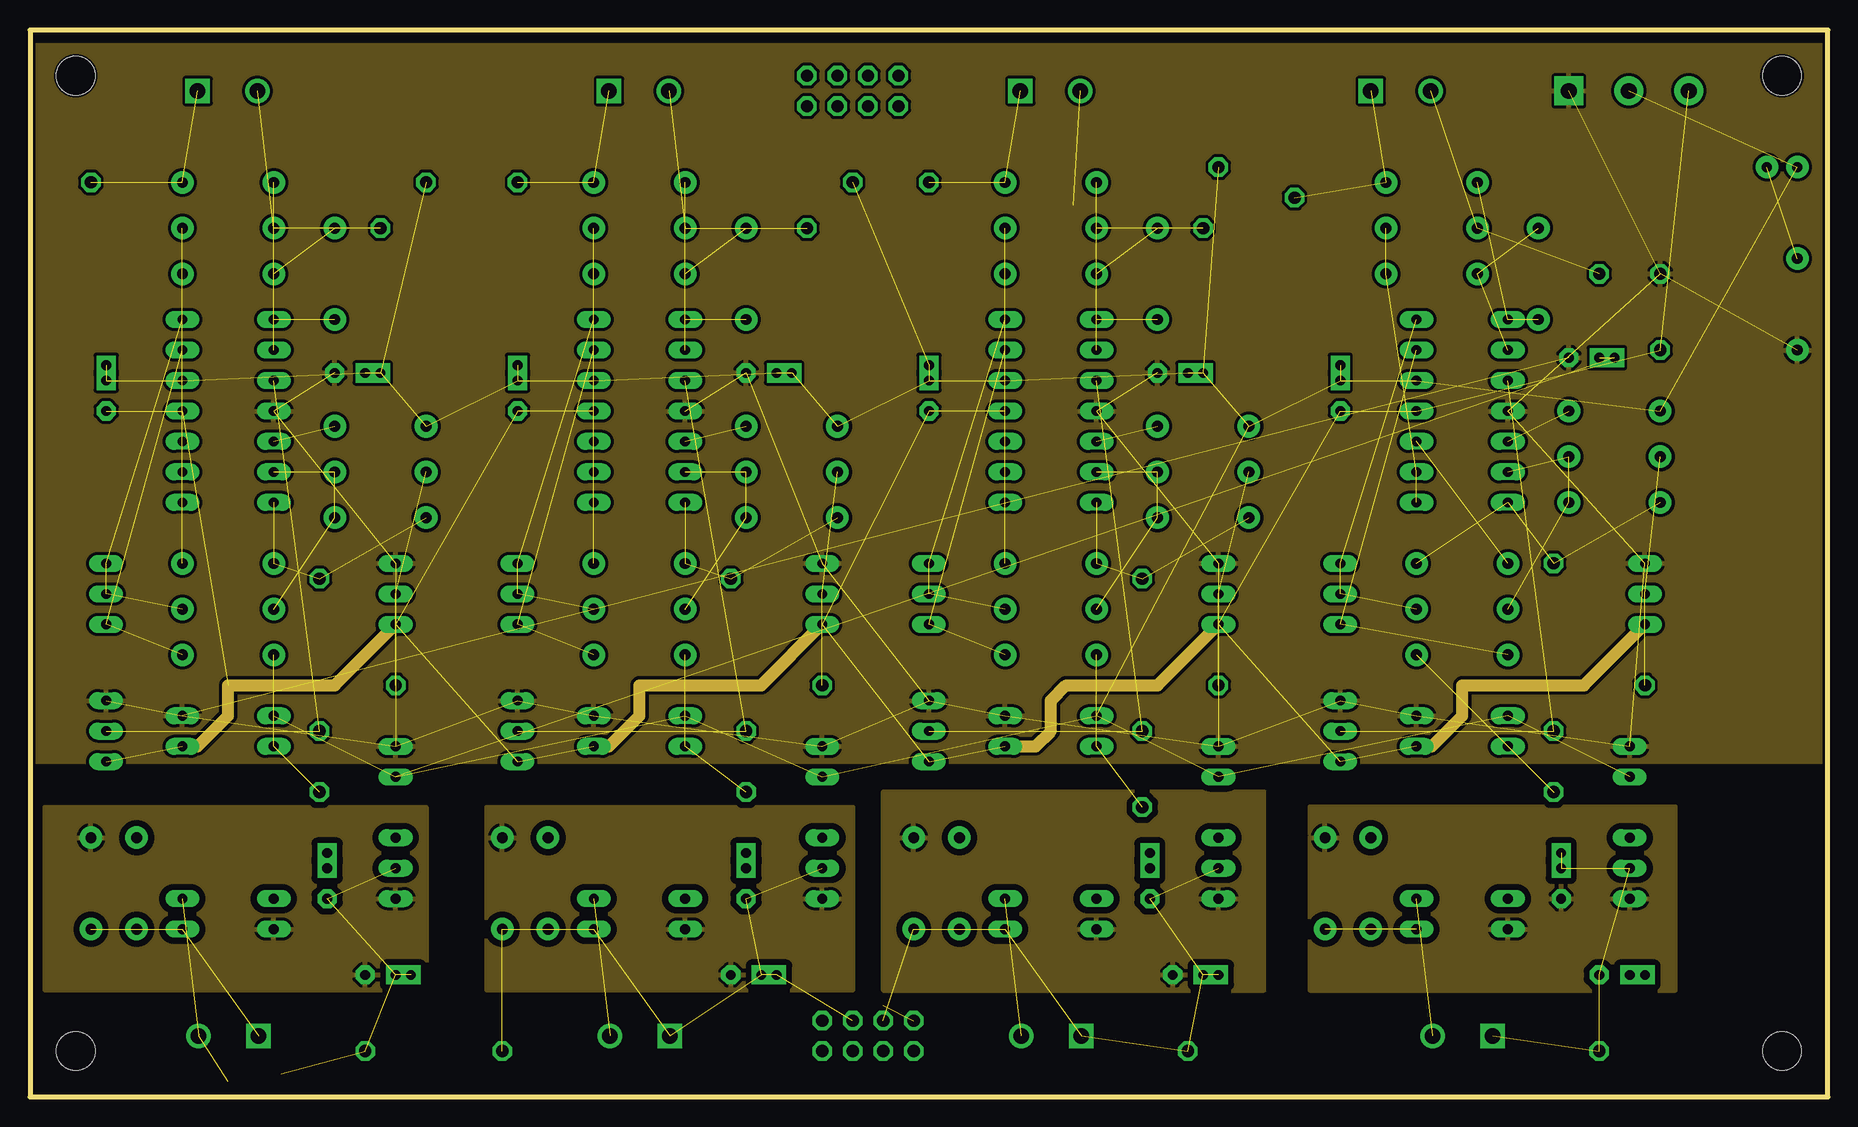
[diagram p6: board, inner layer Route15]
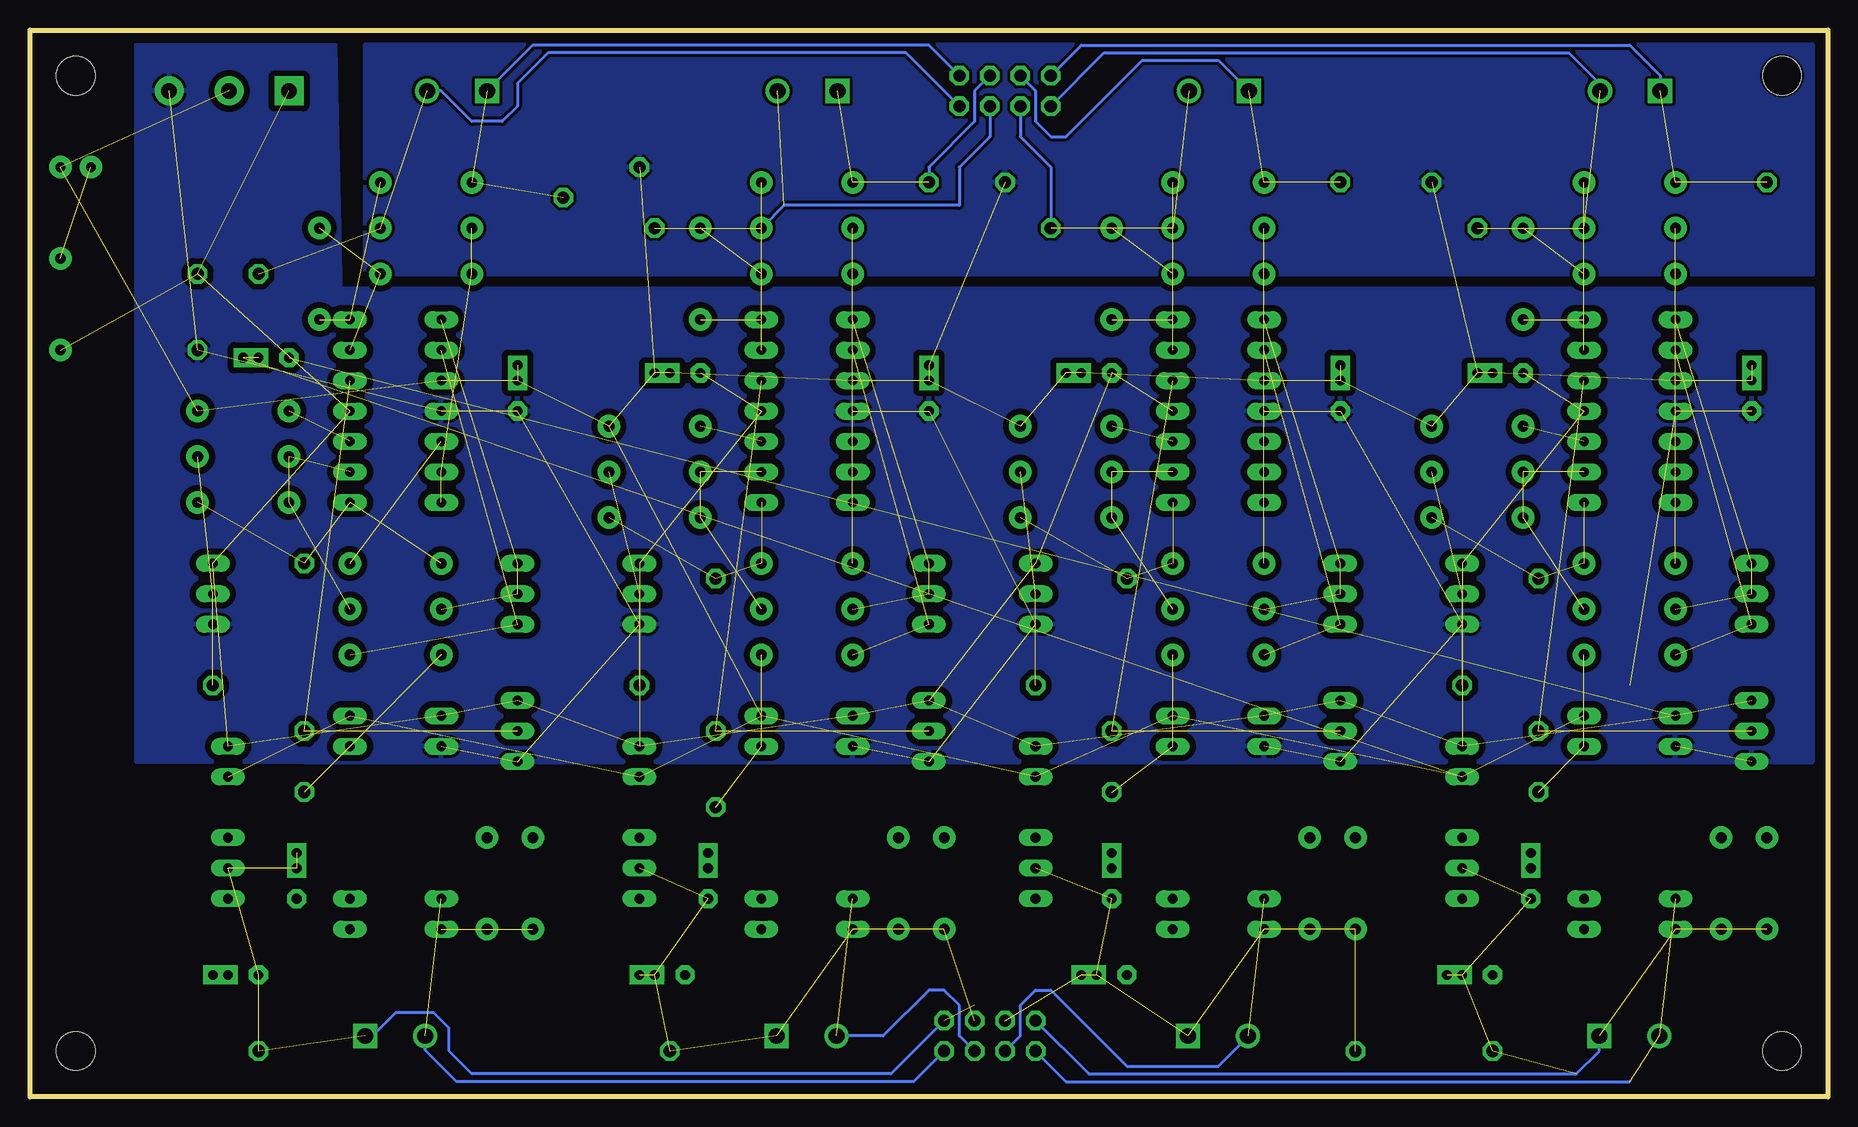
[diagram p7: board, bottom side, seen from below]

Size 149.86 x 88.9 mm. Coordinates in mm from the lower left corner, seen from the top.
Outline: 0,0 149.86,0 149.86,88.9 0,88.9 0,0
Copper layers (1*2*15*16): Top 0.035mm / dielectric 1.5mm / Route2 0.035mm / dielectric 0.15mm / Route15 0.035mm / dielectric 0.2mm / Bottom 0.035mm
Design rules "SeeedStudio_2layer_DRU_no_angle_20140221 *": minimum track width 10mil, minimum drill 20mil, track to track 10mil, track to pad 10mil, pad to pad 10mil, via to via 10mil, smd to smd 8mil, copper to edge 8mil, drill to drill 8mil, minimum pad ring 12mil, minimum via ring 10mil, stop-mask expansion 4mil, vias tented up to drill 25mil, thermal gap 10mil
Holes 3.2 mm at 3.81,85.09 3.81,3.81 146.05,85.09 146.05,3.81

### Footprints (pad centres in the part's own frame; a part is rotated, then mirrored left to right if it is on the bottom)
1X01 = drill 1.016 octagon: 1 0,0
2X04 = drill 1.016 octagon: 1 -3.81,-1.27; 2 -3.81,1.27; 3 -1.27,-1.27; 4 -1.27,1.27; 5 1.27,-1.27; 6 1.27,1.27; 7 3.81,-1.27; 8 3.81,1.27
SCREWTERMINAL-5MM-2 = drill 1.3 pad 2.032 square: 1 0,0 | drill 1.3 pad 2.032: 2 5,0
1+2CAP = drill 0.813 pad 1.6 octagon: 1 -2.54,0 | drill 0.813 pad 1.6 square: 2@1 0,0; 2@2 1.27,0
SIL6-5 = drill 0.813 long: 1 -10.16,0; 2 -7.62,0; 4 -2.54,0; 5 0,0; 6 2.54,0
DIL16-8 = drill 0.813 long: 1 -8.89,-3.81; 2 -6.35,-3.81; 7 6.35,-3.81; 8 8.89,-3.81; 9 8.89,3.81; 10 6.35,3.81; 15 -6.35,3.81; 16 -8.89,3.81
DIL14 = drill 0.813 long: 1 -7.62,-3.81; 2 -5.08,-3.81; 3 -2.54,-3.81; 4 0,-3.81; 5 2.54,-3.81; 6 5.08,-3.81; 7 7.62,-3.81; 8 7.62,3.81; 9 5.08,3.81; 10 2.54,3.81; 11 0,3.81; 12 -2.54,3.81; 13 -5.08,3.81; 14 -7.62,3.81
SCREWTERMINAL-5MM-3 = drill 1.3 pad 2.413 square: 1 0,0 | drill 1.3 pad 2.413: 2 5,0; 3 10,0
LED5MM = drill 0.813 pad 1.88: A -1.27,0; K 1.27,0
AXIAL-0.3 = drill 0.9 pad 1.88: P$1 -3.81,0; P$2 3.81,0
B64Y = drill 0.813 long: A 2.54,0; E -2.54,0; S 0,0

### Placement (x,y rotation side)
+12V  135.89,68.58 0 top
-12V  135.89,62.23 0 top
_GND  99.06,77.47 0 top
AIN  69.85,5.08 0 top
AIN0  19.05,5.08 180 top
AIN1  53.34,5.08 180 top
AIN2  87.63,5.08 180 top
AIN3  121.92,5.08 180 top
AOUT0  13.97,83.82 0 top
AOUT1  48.26,83.82 0 top
AOUT2  82.55,83.82 0 top
AOUT3  111.76,83.82 0 top
C1  30.48,10.16 0 top
C2  24.77,19.05 90 top
C3  6.35,59.69 90 top
C4  59.69,19.05 90 top
C5  60.96,10.16 0 top
C6  40.64,59.69 90 top
C7  93.34,19.05 90 top
C8  97.79,10.16 0 top
C9  74.93,59.69 90 top
C10  133.35,10.16 0 top
C11  127.64,19.05 90 top
C12  109.22,59.69 90 top
C13  27.94,60.33 0 top
C14  62.23,60.33 0 top
C15  96.52,60.33 0 top
C16  130.81,61.59 0 top
FRAME1  114.3,1.27 0 top
FRAME2  114.3,2.54 90 top
FRAME3  not placed on the board
FRAME4  not placed on the board
GND  33.02,76.2 0 top
GND_  68.58,76.2 0 top
GND_0  27.94,3.81 0 top
GND_1  39.37,3.81 0 top
GND_2  96.52,3.81 0 top
GND_3  130.81,3.81 0 top
IC1_0  30.48,19.05 270 top
IC1_1  66.04,19.05 270 top
IC1_2  99.06,19.05 270 top
IC1_3  133.35,19.05 270 top
IC2_0  16.51,22.86 90 top
IC2_1  50.8,22.86 90 top
IC2_2  85.09,22.86 90 top
IC2_3  119.38,22.86 90 top
IC3_0  16.51,57.15 90 top
IC3_1  50.8,57.15 90 top
IC3_2  85.09,57.15 90 top
IC3_3  119.38,57.15 90 top
J7  128.27,83.82 0 top
PPAIO16/4  68.58,83.82 0 top
PWR  146.05,77.47 0 top
R1_0  16.51,36.83 180 top
R1_1  50.8,36.83 180 top
R1_2  85.09,36.83 180 top
R1_3  119.38,36.83 0 top
R4_0  16.51,40.64 0 top
R4_1  50.8,40.64 0 top
R4_2  85.09,40.64 0 top
R4_3  119.38,40.64 0 top
R5_0  29.21,52.07 180 top
R5_1  63.5,52.07 180 top
R5_2  97.79,52.07 180 top
R5_3  132.08,53.34 180 top
R6_0  29.21,48.26 0 top
R6_1  63.5,48.26 0 top
R6_2  97.79,48.26 0 top
R6_3  132.08,49.53 0 top
R7_0  29.21,55.88 180 top
R7_1  63.5,55.88 180 top
R7_2  97.79,55.88 180 top
R7_3  132.08,57.15 180 top
R8_0  16.51,44.45 180 top
R8_1  50.8,44.45 180 top
R8_2  85.09,44.45 180 top
R8_3  119.38,44.45 0 top
R9_0  16.51,72.39 0 top
R9_1  50.8,72.39 0 top
R9_2  85.09,72.39 0 top
R9_3  116.84,72.39 0 top
R10_0  25.4,68.58 270 top
R10_1  59.69,68.58 270 top
R10_2  93.98,68.58 270 top
R10_3  125.73,68.58 270 top
R11_0  16.51,68.58 0 top
R11_1  50.8,68.58 0 top
R11_2  85.09,68.58 0 top
R11_3  116.84,68.58 0 top
R12_0  16.51,76.2 180 top
R12_1  50.8,76.2 180 top
R12_2  85.09,76.2 180 top
R12_3  116.84,76.2 180 top
R19_0  8.89,17.78 90 top
R19_1  43.18,17.78 90 top
R19_2  77.47,17.78 90 top
R19_3  111.76,17.78 90 top
R20_0  5.08,17.78 90 top
R20_1  39.37,17.78 90 top
R20_2  73.66,17.78 90 top
R20_3  107.95,17.78 90 top
R24  147.32,66.04 270 top
SPAN  6.35,41.91 270 top
SPAN1  40.64,41.91 270 top
SPAN2  74.93,41.91 270 top
SPAN3  109.22,41.91 270 top
TP1_0  24.13,25.4 0 top
TP1_1  59.69,25.4 0 top
TP1_2  92.71,24.13 0 top
TP1_3  127,25.4 0 top
TP3_0  30.48,34.29 0 top
TP3_1  66.04,34.29 0 top
TP3_2  99.06,34.29 0 top
TP3_3  134.62,34.29 0 top
TP4_0  24.13,43.18 0 top
TP4_1  58.42,43.18 0 top
TP4_2  92.71,43.18 0 top
TP4_3  127,44.45 0 top
TP5_0  29.21,72.39 0 top
TP5_1  64.77,72.39 0 top
TP5_2  97.79,72.39 0 top
TP5_3  130.81,68.58 0 top
TP6_0  5.08,76.2 0 top
TP6_1  40.64,76.2 0 top
TP6_2  74.93,76.2 0 top
TP6_3  105.41,74.93 0 top
TP7_0  24.13,30.48 0 top
TP7_1  59.69,30.48 0 top
TP7_2  92.71,30.48 0 top
TP7_3  127,30.48 0 top
VREF  6.35,30.48 270 top
VREF1  40.64,30.48 270 top
VREF2  74.93,30.48 270 top
VREF3  109.22,30.48 270 top
ZERO  30.48,41.91 270 top
ZERO1  66.04,41.91 270 top
ZERO2  99.06,41.91 270 top
ZERO3  134.62,41.91 270 top

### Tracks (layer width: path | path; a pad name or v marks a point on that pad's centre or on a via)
+12_0
  pour Route15: 1.27,24.13 33.02,24.13 33.02,8.89 1.27,8.89
+12_1
  pour Route15: 38.1,24.13 68.58,24.13 68.58,8.89 38.1,8.89
+12_2
  pour Route15: 71.12,8.89 102.87,8.89 102.87,25.4 71.12,25.4
+12_3
  pour Route15: 106.68,8.89 137.16,8.89 137.16,24.13 106.68,24.13
+12V  (26 unrouted)
  pour Route15: 0,87.63 149.86,87.63 149.86,27.94 0,27.94
-12_0
  pour Top: 1.27,24.13 33.02,24.13 33.02,8.89 1.27,8.89
-12_1
  pour Top: 38.1,24.13 68.58,24.13 68.58,8.89 38.1,8.89
-12_2
  pour Top: 71.12,8.89 101.6,8.89 101.6,24.13 71.12,24.13
-12_3
  pour Top: 105.41,8.89 137.16,8.89 137.16,24.13 105.41,24.13
-12V  (17 unrouted)
  Top 1.016: IC2_0.10 13.97,29.21 16.51,31.75 16.51,33.02 17.78,34.29 25.4,34.29 ZERO.A | IC2_1.10 49.53,29.21 50.8,30.48 50.8,33.02 52.07,34.29 60.96,34.29 ZERO1.A | IC2_2.10 83.82,29.21 85.09,30.48 85.09,33.02 86.36,34.29 93.98,34.29 ZERO2.A | IC2_3.10 118.11,29.21 119.38,30.48 119.38,33.02 120.65,34.29 129.54,34.29 ZERO3.A
  Route2 1.016: IC2_0.10 13.97,29.21 16.51,31.75 16.51,34.29 25.4,34.29 ZERO.A | IC2_1.10 49.53,29.21 50.8,30.48 50.8,33.02 52.07,34.29 60.96,34.29 ZERO1.A | IC2_2.10 82.55,29.21 87.63,34.29 93.98,34.29 ZERO2.A | IC2_3.10 118.11,29.21 119.38,30.48 119.38,33.02 120.65,34.29 129.54,34.29 ZERO3.A
  Route15 1.016: IC2_3.10 116.84,29.21 119.38,31.75 119.38,34.29 129.54,34.29 ZERO3.A | IC2_2.10 83.82,29.21 85.09,30.48 85.09,33.02 86.36,34.29 93.98,34.29 ZERO2.A | IC2_1.10 48.26,29.21 50.8,31.75 50.8,34.29 60.96,34.29 ZERO1.A | IC2_0.10 13.97,29.21 16.51,31.75 16.51,34.29 25.4,34.29 ZERO.A
  pour Bottom: 1.27,67.31 127,67.31 127,27.94 1.27,27.94
  pour Bottom: 124.46,87.63 123.19,27.94 140.97,27.94 140.97,87.63
AIN0+  (2 unrouted)
  Bottom 0.254: AIN.1 63.5,1.27 16.51,1.27
AIN1+  (1 unrouted)
  Bottom 0.254: AIN.3 67.31,5.08 67.31,7.62 66.04,8.89 64.77,8.89 58.42,2.54 50.8,2.54 48.34,5 AIN1.2
AIN2+  (1 unrouted)
  Bottom 0.254: AIN.5 72.39,5.08 72.39,7.62 73.66,8.89 74.93,8.89 78.74,5.08 AIN2.2
AIN3+  (1 unrouted)
  Bottom 0.254: AIN.7 76.2,1.27 114.3,1.27 116.92,3.89 AIN3.2
AOUT0+  (2 unrouted)
  Bottom 0.254: PPAIO16/4.1 60.33,87 21.59,87 18.97,84.38 AOUT0.2
AOUT0-  (2 unrouted)
  Bottom 0.254: PPAIO16/4.2 62.23,87.63 16.51,87.63 13.97,85.09 AOUT0.1
AOUT1+  (2 unrouted)
  Bottom 0.254: PPAIO16/4.3 67.31,80.01 64.77,77.47 TP5_1.1
AOUT1-  (2 unrouted)
  Bottom 0.254: PPAIO16/4.4 66.04,83.82 66.04,81.28 64.77,80.01 63.5,80.01 57.15,86.36 50.8,86.36 AOUT1.1
AOUT2+  (2 unrouted)
  Bottom 0.254: PPAIO16/4.5 69.85,80.01 72.39,77.47 72.39,74.3 87,74.3 R9_2.P$2
AOUT2-  (2 unrouted)
  Bottom 0.254: PPAIO16/4.6 71.12,83.82 71.12,81.28 74.93,77.47 TP6_2.1
AOUT3+  (2 unrouted)
  Bottom 0.254: PPAIO16/4.7 76.83,87 106.68,87 109.22,84.45 109.22,82.55 110.49,81.28 113.03,81.28 115.57,83.82 AOUT3.2
AOUT3-  (2 unrouted)
  Bottom 0.254: PPAIO16/4.8 74.93,87.63 107.95,87.63 AOUT3.1
GND  (36 unrouted)
  pour Route2: 1.27,87.63 149.86,87.63 149.86,25.4 1.27,25.4
  pour Bottom: 1.27,87.63 121.92,87.63 121.92,68.58 1.27,68.58
  pour Top: 1.27,87.63 129.54,87.63 129.54,27.94 1.27,27.94
  pour Top: 109.22,87.63 142.24,87.63 142.24,60.96 109.22,60.96
GND0  (8 unrouted)
  Bottom 0.254: AIN.2 61.59,1.91 20.95,1.91 19.05,3.81 AIN0.1
  pour Route2: 1.27,22.86 33.02,22.86 33.02,0 1.27,0
GND1  (9 unrouted)
  pour Route2: 38.1,22.86 68.58,22.86 68.58,0 38.1,0
GND2  (9 unrouted)
  pour Route2: 71.12,22.86 101.6,22.86 101.6,0 71.12,0
GND3  (8 unrouted)
  Top 0.406: 71.12,7.62 72.39,8.89 91.44,8.89 93.98,6.35 105.41,6.35 106.68,7.62 106.68,12.7 R20_3.P$1
  Bottom 0.254: AIN.8 78.11,1.91 113.03,1.91 114.94,3.81 114.94,5.71 116.2,6.99 119.38,6.99 121.28,5.08 AIN3.1
  pour Route2: 104.14,22.86 135.89,22.86 135.89,0 104.14,0
N$1  (2 unrouted)
N$2  (1 unrouted)
N$3  (3 unrouted)
N$4  (3 unrouted)
N$5  (3 unrouted)
N$6  (2 unrouted)
N$8  (2 unrouted)
N$9  (1 unrouted)
N$10  (2 unrouted)
N$11  (3 unrouted)
N$12  (2 unrouted)
N$13  (2 unrouted)
N$17  (2 unrouted)
N$18  (3 unrouted)
N$19  (3 unrouted)
N$20  (3 unrouted)
N$22  (2 unrouted)
N$23  (2 unrouted)
N$24  (1 unrouted)
N$26  (1 unrouted)
N$29  (2 unrouted)
N$30  (1 unrouted)
N$31  (3 unrouted)
N$32  (2 unrouted)
N$33  (2 unrouted)
N$34  (2 unrouted)
N$35  (3 unrouted)
N$36  (3 unrouted)
N$37  (3 unrouted)
N$39  (2 unrouted)
N$40  (2 unrouted)
N$41  (1 unrouted)
N$45  (2 unrouted)
N$46  (1 unrouted)
N$47  (3 unrouted)
N$48  (2 unrouted)
N$49  (2 unrouted)
N$50  (2 unrouted)
N$51  (3 unrouted)
N$52  (3 unrouted)
N$53  (3 unrouted)
N$55  (2 unrouted)
N$56  (2 unrouted)
N$57  (1 unrouted)
N$61  (2 unrouted)
N$62  (1 unrouted)
N$63  (3 unrouted)
N$64  (2 unrouted)
N$65  (2 unrouted)

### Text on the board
tPlace: 1 | -Aout0+ | -Aout1+ | -Aout2+ | -Aout3+ | + Gnd - | 12V | Rev 1 | PPAC4 / 4-Ch Analog Conditioning / Copyright 2017 / Plantation Productions, Inc. | +Ain0- | +Ain1- | +Ain2- | +Ain3- | REV 2 | 1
